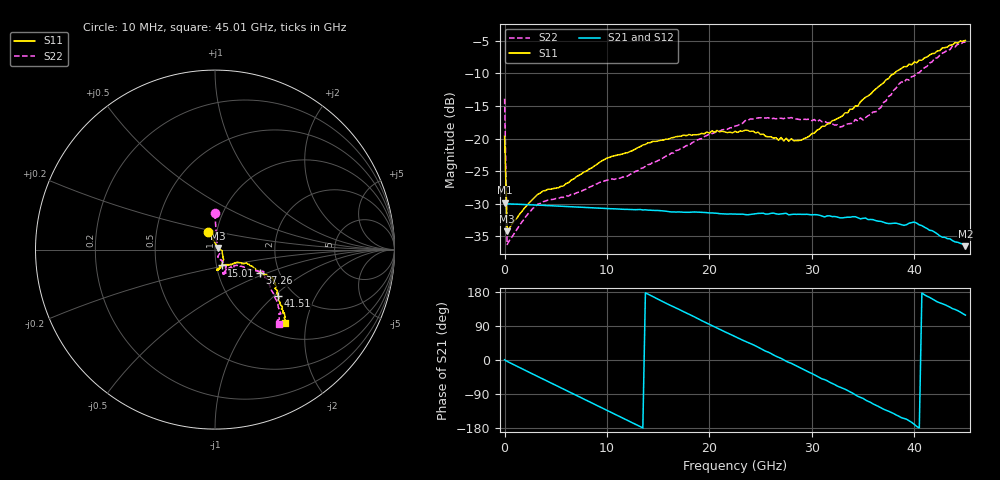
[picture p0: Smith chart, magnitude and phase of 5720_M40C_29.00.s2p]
! Device:  ADRF5720
! Description: 0.5dB LSB GaAs MMIC 6-bit Digital Attenuator
! Frequency:  0.000009 -  40 GHz
! Ports:
!	RF1	= Port 1
!	RF2	= Port 2
! Vdd:  3.3 Volt
! Vss:  -3.3 Volt
! Control:  0/3.3 Volt
! State:  29.00 dB attenuation
! Data:  The device was measured using G-S-G Probes on a matrix board.
!  Data was collected using an calibrated 4 port network analyzer.
!  The reference plane for this measurement is at the launchers.
! Note:  Analog Devices supplies this data as a sample of measured data
!  for this product.  Your particular data for this product may vary.
!  Data was taken at -40 degrees C.
!  Analog Devices reserves the right to change this data at anytime.
# GHZ S DB R 45.0
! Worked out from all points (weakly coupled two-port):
!   181 points, 10 MHz to 45.01 GHz, reference 45 ohm
!   highest |S21| = -29.84 dB at 10 MHz (marker M1); lowest = -36.5 dB at 45.01 GHz (marker M2)
!   lowest |S11| = -34.2 dB at 260 MHz (marker M3), VSWR 1.04, Z = 46.5 + j0.9 ohm
!   |S11| at or under -10 dB: start of sweep to 38.08 GHz
!   |S22| runs from -36.2 to -5.2 dB; largest |S21 - S12| = 0.00016
!   S11 on the Smith chart (normalised r, x): 10 MHz: 0.91, +0.18; 15.01 GHz: 1.06, -0.19; 37.26 GHz: 1.59, -0.45; 41.51 GHz: 1.67, -1.06; 45.01 GHz: 1.27, -1.52
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0.01  -19.64 110.8  -29.84 0.5  -29.86 0.4  -13.89 90.3
0.26  -34.21 29.7  -30.02 -3.6  -30.04 -3.7  -36.24 32.4
3.26  -28.54 -7.6  -30.21 -43.7  -30.24 -43.8  -30.07 -32.6
5.76  -27.27 -23.4  -30.39 -76.6  -30.42 -76.6  -29.02 -52.6
7.76  -25.14 -37.8  -30.55 -102.9  -30.57 -103.0  -27.87 -65.8
10.01  -22.98 -47.9  -30.73 -132.7  -30.75 -132.7  -26.39 -67.5
12.01  -22.17 -56.5  -30.86 -159.1  -30.88 -159.2  -25.77 -66.0
15.01  -20.37 -67.2  -31.03 160.3  -31.05 160.3  -23.36 -59.4
15.26  -20.26 -68.3  -31.06 156.7  -31.07 156.7  -23.20 -59.6
20.26  -18.82 -81.6  -31.41 90.6  -31.44 90.5  -19.24 -57.8
22.76  -19.06 -85.2  -31.59 58.8  -31.61 58.7  -18.00 -63.4
24.01  -18.92 -80.7  -31.64 43.6  -31.67 43.5  -16.99 -64.7
27.76  -20.40 -68.2  -31.70 -6.3  -31.71 -6.4  -16.86 -69.0
30.26  -19.17 -48.7  -31.67 -39.0  -31.70 -39.1  -17.09 -70.4
33.01  -16.53 -28.6  -32.16 -73.9  -32.19 -74.0  -18.15 -55.5
35.01  -14.01 -24.2  -32.23 -101.2  -32.25 -101.3  -17.15 -40.2
37.26  -10.99 -27.6  -32.97 -132.6  -33.01 -132.8  -14.23 -31.6
37.76  -10.28 -27.1  -33.03 -138.2  -33.05 -138.3  -13.29 -30.2
38.51  -9.49 -26.9  -33.09 -148.4  -33.11 -148.7  -11.66 -26.8
39.76  -8.70 -27.9  -32.89 -164.5  -32.92 -164.6  -10.52 -24.2
41.51  -7.20 -36.1  -34.06 165.4  -34.08 165.3  -8.45 -34.7
45.01  -4.97 -46.2  -36.50 118.6  -36.48 118.6  -5.23 -49.6
